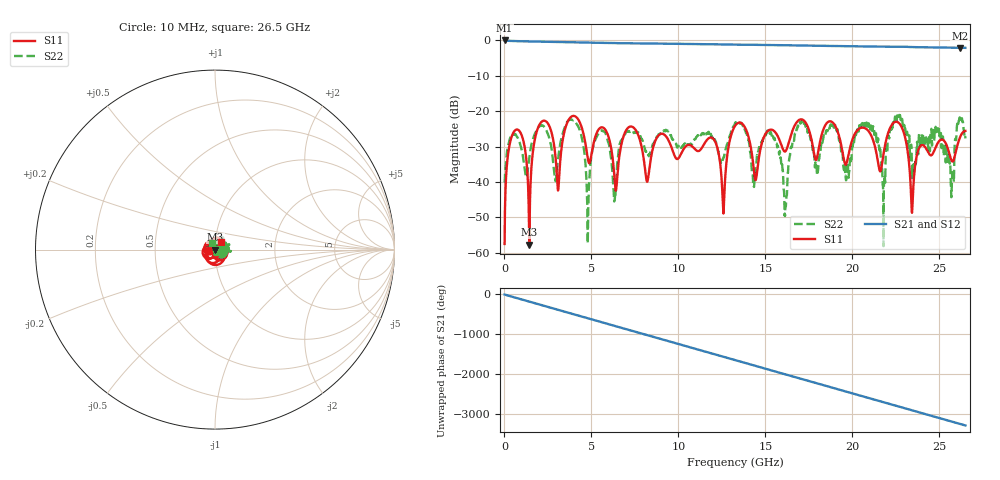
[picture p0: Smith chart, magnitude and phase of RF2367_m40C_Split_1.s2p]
!Keysight Technologies,N5245B,MY55451909,A.13.80.08
!Automatic Fixture Removal (AFR)
!Date: Thursday, August 27, 2020, 03:56:56
!S2P File: Measurements: S11,S21,S12,S22:
# MHz S  RI  R 50
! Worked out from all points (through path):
!   2650 points, 10 MHz to 26.5 GHz, reference 50 ohm
!   highest |S21| = 0.00 dB at 10 MHz (marker M1); lowest = -2.1 dB at 26.17 GHz (marker M2)
!   group delay of S21, straight-line fit = 345 ps
!   lowest |S11| = -57.7 dB at 1.43 GHz (marker M3), VSWR 1.00, Z = 50.1 - j0.00338 ohm
!   |S11| at or under -10 dB: start of sweep to end of sweep
!   |S22| runs from -58.1 to -21.0 dB; largest |S21 - S12| = 1.4e-15
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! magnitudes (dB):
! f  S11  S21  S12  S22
! 10 MHz  -57.5  0.0  0.0  -40.1
! 610 MHz  -25.4  -0.2  -0.2  -26.4
! 1.43 GHz  -57.7  -0.3  -0.3  -33.2
! 2.09 GHz  -23.2  -0.4  -0.4  -24.1
! 3.08 GHz  -42.4  -0.5  -0.5  -33.8
! 4.43 GHz  -24.4  -0.6  -0.6  -27.1
! 4.8 GHz  -33.5  -0.6  -0.6  -53.4
! 5.5 GHz  -24.7  -0.7  -0.7  -25.6
! 6.33 GHz  -39.0  -0.7  -0.7  -45.2
! 8.84 GHz  -26.9  -0.9  -0.9  -26.8
! 11.98 GHz  -27.7  -1.1  -1.1  -27.6
! 12.58 GHz  -48.7  -1.1  -1.1  -33.4
! 13.26 GHz  -24.1  -1.2  -1.2  -23.3
! 16.15 GHz  -31.3  -1.4  -1.4  -47.1
! 16.87 GHz  -22.7  -1.4  -1.4  -24.0
! 17.67 GHz  -28.4  -1.5  -1.5  -29.4
! 21.78 GHz  -32.5  -1.8  -1.8  -46.7
! 22.09 GHz  -25.7  -1.8  -1.8  -26.9
! 23.44 GHz  -48.3  -1.9  -1.9  -38.9
! 25.73 GHz  -34.1  -2.1  -2.1  -39.0
! 26.17 GHz  -27.6  -2.1  -2.1  -21.8
! 26.5 GHz  -25.6  -2.1  -2.1  -27.7
